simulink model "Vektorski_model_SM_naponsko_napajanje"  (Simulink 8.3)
settings: Solver=ode3  StartTime=0  StopTime=Tfinal  FixedStep=Tsim  RelTol=1e-3
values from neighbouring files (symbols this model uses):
  A1 = [-Rs/Ld 0; 0 -Rs/Lq]    [Vektorski_model_SM_naponsko_napajanje_parametri.m]
  A2 = [0 Lq/Ld; -Ld/Lq 0]    [Vektorski_model_SM_naponsko_napajanje_parametri.m]
  Am = [-Kfv*p/J -Kel*p/J; 1 0]    [Vektorski_model_SM_naponsko_napajanje_parametri.m]
  B = [1/Ld 0; 0 1/Lq]    [Vektorski_model_SM_naponsko_napajanje_parametri.m]
  Bm = [p/J -p/J; 0 0]    [Vektorski_model_SM_naponsko_napajanje_parametri.m]
  Ids_ref = 0    [Vektorski_model_SM_naponsko_napajanje_parametri.m]
  Iqs_ref = 1    [Vektorski_model_SM_naponsko_napajanje_parametri.m]
  Ki = lambda*Rs    [Vektorski_model_SM_naponsko_napajanje_parametri.m]
  Kpd = lambda*Ld    [Vektorski_model_SM_naponsko_napajanje_parametri.m]
  Kpq = lambda*Lq    [Vektorski_model_SM_naponsko_napajanje_parametri.m]
  L = [Ld 0; 0 Lq]    [Vektorski_model_SM_naponsko_napajanje_parametri.m]
  Ld = 0.0370    (= 0.037)    [Vektorski_model_SM_naponsko_napajanje_parametri.m]
  Lq = 0.0485    [Vektorski_model_SM_naponsko_napajanje_parametri.m]
  Mopt = 2    [Vektorski_model_SM_naponsko_napajanje_parametri.m]
  p = 5    [Vektorski_model_SM_naponsko_napajanje_parametri.m]
  PSI = 0.1345    [Vektorski_model_SM_naponsko_napajanje_parametri.m]
  topt = 1    [Vektorski_model_SM_naponsko_napajanje_parametri.m]
  Tsim = Tpwm/16    (= 3.125e-06)    [Vektorski_model_SM_naponsko_napajanje_parametri.m]
libraries: simulink x1

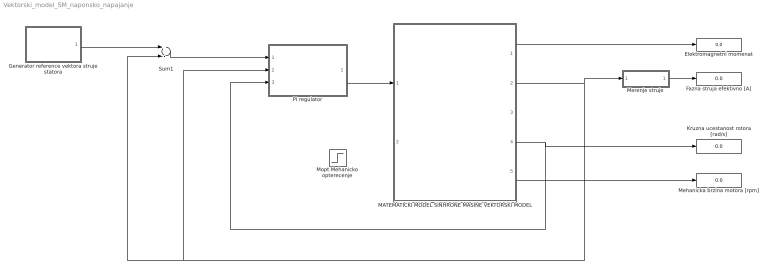
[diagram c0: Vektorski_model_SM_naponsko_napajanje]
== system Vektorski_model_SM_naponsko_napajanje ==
  Elektromagnetni momenat : Display
  Fazna struja efektivno [A] : Display
  Generator reference vektora struje statora : Subsystem
  Kruzna ucestanost rotora [rad/s] : Display
  MATEMATICKI MODEL SINHRONE MASINE VEKTORSKI MODEL : Subsystem
  Mehanicka brzina motora [rpm] : Display
  Merenje struje : Subsystem
  Mopt Mehanicko opterecenje : Step  Time=4*topt  After=Mopt  SampleTime=Tsim
  PI regulator : Subsystem
  Sum1 : Sum  Inputs=+-  SampleTime=Tsim
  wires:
  MATEMATICKI MODEL SINHRONE MASINE VEKTORSKI MODEL/1(M_el) -> Elektromagnetni momenat/1
  MATEMATICKI MODEL SINHRONE MASINE VEKTORSKI MODEL/5(Brzina meh [o/min]) -> Mehanicka brzina motora [rpm]/1
  Merenje struje/1(Is_eff) -> Fazna struja efektivno [A]/1
  MATEMATICKI MODEL SINHRONE MASINE VEKTORSKI MODEL/4(wr_el) -> PI regulator/3(w), Kruzna ucestanost rotora [rad/s]/1
  MATEMATICKI MODEL SINHRONE MASINE VEKTORSKI MODEL/2(Is) -> Merenje struje/1(Is_dq), Sum1/2, PI regulator/2(Is)
  Sum1/1 -> PI regulator/1(e)
  PI regulator/1(Us_ref) -> MATEMATICKI MODEL SINHRONE MASINE VEKTORSKI MODEL/1(Us_dq)
  Generator reference vektora struje statora/1(Is_ref) -> Sum1/1

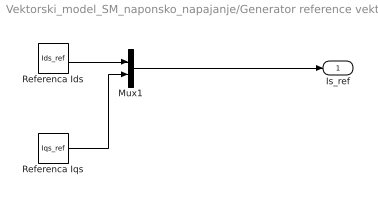
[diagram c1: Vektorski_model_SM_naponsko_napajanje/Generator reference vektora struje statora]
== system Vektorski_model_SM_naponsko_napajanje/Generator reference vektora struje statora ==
  Mux1 : Mux  Inputs=2
  Referenca Ids : Constant  Value=Ids_ref  SampleTime=Tsim
  Referenca Iqs : Constant  Value=Iqs_ref  SampleTime=Tsim
  Is_ref : Outport
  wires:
  Mux1/1 -> Is_ref/1
  Referenca Ids/1 -> Mux1/1
  Referenca Iqs/1 -> Mux1/2

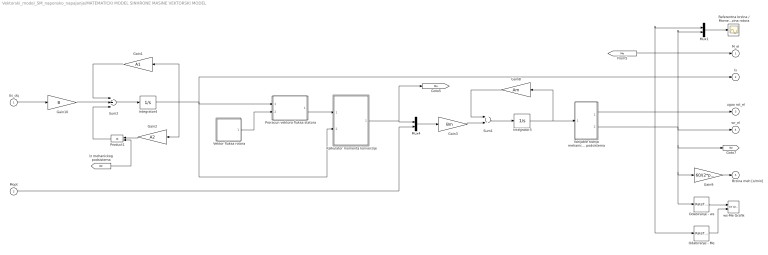
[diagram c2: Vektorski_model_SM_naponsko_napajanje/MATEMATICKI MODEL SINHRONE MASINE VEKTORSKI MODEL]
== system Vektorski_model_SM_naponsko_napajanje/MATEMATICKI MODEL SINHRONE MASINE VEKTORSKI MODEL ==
  Us_dq : Inport
  Mopt : Inport  Port=2
  Gain1 : Gain  Gain=A1  Multiplication=Matrix(K*u) (u vector)  SampleTime=Tsim
  Gain10 : Gain  Gain=B  Multiplication=Matrix(K*u) (u vector)  SampleTime=Tsim
  Gain2 : Gain  Gain=A2  Multiplication=Matrix(K*u) (u vector)  SampleTime=Tsim
  Gain3 : Gain  Gain=Bm  Multiplication=Matrix(K*u) (u vector)  SampleTime=Tsim
  Gain8 : Gain  Gain=Am  Multiplication=Matrix(K*u) (u vector)  SampleTime=Tsim
  Gain9 : Gain  Gain=60/(2*pi()*p)  SampleTime=Tsim
  Integrator3 : Integrator  InitialCondition=[0,0]
  Integrator4 : Integrator  InitialCondition=[0,0]
  Kalkulator momenta konverzije : Subsystem
  Mux1 : Mux  Inputs=2
  Mux4 : Mux  Inputs=2
  Odabiranje - Me : RateTransition  OutPortSampleTime=100*Tsim
  Odabiranje - ws : RateTransition  OutPortSampleTime=100*Tsim
  Product1 : Product  SampleTime=Tsim
  Proracun vektora fluksa statora : Subsystem
  Referentna brzina / Momenat / Brzina rotora : Scope
  Sum1 : Sum  SampleTime=Tsim
  Sum2 : Sum  Inputs=+++  SampleTime=Tsim
  Varijable stanja mehanickog podsistema : Subsystem
  Vektor fluksa rotora : Subsystem
  ws-Me Grafik : simulink/Sinks/XY Graph  xmin=-400  xmax=400  ymin=-20  ymax=20  st=100*Tsim
  M_el : Outport  InitialOutput=0
  Is : Outport  Port=2  InitialOutput=0
  ugao rot_el : Outport  Port=3  InitialOutput=0
  wr_el : Outport  Port=4  InitialOutput=0
  Brzina meh [o/min] : Outport  Port=5  InitialOutput=0
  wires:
  Kalkulator momenta konverzije/1(Me) -> [Me], Mux4/1
  Mopt/1 -> Mux4/2
  [Me] -> Mux1/1, M_el/1, Odabiranje - Me/1
  Varijable stanja mehanickog podsistema/1(theta) -> ugao rot_el/1
  Varijable stanja mehanickog podsistema/2(w) -> Mux1/2, Odabiranje - ws/1, Gain9/1, [Wr], wr_el/1
  Gain9/1 -> Brzina meh [o/min]/1
  Mux4/1 -> Gain3/1
  Gain3/1 -> Sum1/2
  Sum1/1 -> Integrator3/1
  Gain8/1 -> Sum1/1
  Integrator3/1 -> Varijable stanja mehanickog podsistema/1(X2), Gain8/1
  Mux1/1 -> Referentna brzina / Momenat / Brzina rotora/1
  Odabiranje - ws/1 -> ws-Me Grafik/1
  Odabiranje - Me/1 -> ws-Me Grafik/2
  Sum2/1 -> Integrator4/1
  Gain2/1 -> Product1/1
  Integrator4/1 -> Kalkulator momenta konverzije/2(Is), Is/1, Proracun vektora fluksa statora/1(Is), Gain2/1, Gain1/1
  [Wr] -> Product1/2
  Gain1/1 -> Sum2/1
  Product1/1 -> Sum2/3
  Gain10/1 -> Sum2/2
  Us_dq/1 -> Gain10/1
  Proracun vektora fluksa statora/1(PSIs) -> Kalkulator momenta konverzije/1(PSIs)
  Vektor fluksa rotora/1("[PSIpm 0]") -> Proracun vektora fluksa statora/2(PSIr)

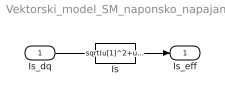
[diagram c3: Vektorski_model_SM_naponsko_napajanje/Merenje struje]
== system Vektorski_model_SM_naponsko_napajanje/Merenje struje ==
  Is_dq : Inport
  Is : Fcn  Expr=sqrt(u[1]^2+u[2]^2)  SampleTime=Tsim
  Is_eff : Outport
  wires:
  Is_dq/1 -> Is/1
  Is/1 -> Is_eff/1

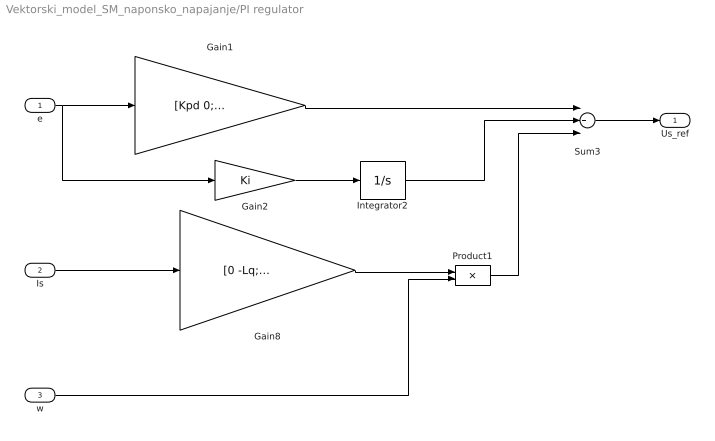
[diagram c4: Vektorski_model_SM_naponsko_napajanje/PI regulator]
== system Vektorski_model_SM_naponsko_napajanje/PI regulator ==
  e : Inport
  Is : Inport  Port=2
  w : Inport  Port=3
  Gain1 : Gain  Gain=[Kpd 0; 0 Kpq]  Multiplication=Matrix(K*u) (u vector)  SampleTime=Tsim
  Gain2 : Gain  Gain=Ki  SampleTime=Tsim
  Gain8 : Gain  Gain=[0 -Lq; Ld 0]  Multiplication=Matrix(K*u) (u vector)  SampleTime=Tsim
  Integrator2 : Integrator  InitialCondition=[0,0]
  Product1 : Product  SampleTime=Tsim
  Sum3 : Sum  Inputs=+++  SampleTime=Tsim
  Us_ref : Outport
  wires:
  Sum3/1 -> Us_ref/1
  Gain2/1 -> Integrator2/1
  Integrator2/1 -> Sum3/2
  e/1 -> Gain2/1, Gain1/1
  Gain1/1 -> Sum3/1
  Is/1 -> Gain8/1
  Gain8/1 -> Product1/1
  w/1 -> Product1/2
  Product1/1 -> Sum3/3

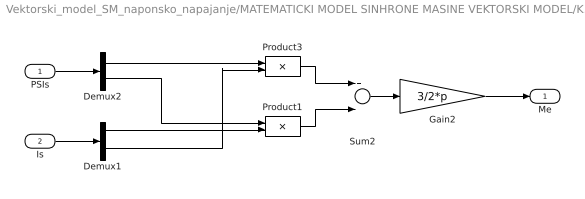
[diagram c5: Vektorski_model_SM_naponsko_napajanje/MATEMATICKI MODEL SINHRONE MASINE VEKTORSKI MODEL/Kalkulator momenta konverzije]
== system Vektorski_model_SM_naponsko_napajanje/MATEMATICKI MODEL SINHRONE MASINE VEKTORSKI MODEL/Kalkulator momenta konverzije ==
  PSIs : Inport
  Is : Inport  Port=2
  Demux1 : Demux  Outputs=2
  Demux2 : Demux  Outputs=2
  Gain2 : Gain  Gain=3/2*p  SampleTime=Tsim
  Product1 : Product  SampleTime=Tsim
  Product3 : Product  SampleTime=Tsim
  Sum2 : Sum  Inputs=+-  SampleTime=Tsim
  Me : Outport
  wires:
  Sum2/1 -> Gain2/1
  Gain2/1 -> Me/1
  Product1/1 -> Sum2/2
  Product3/1 -> Sum2/1
  Demux2/1 -> Product3/1
  Demux2/2 -> Product1/1
  Is/1 -> Demux1/1
  Demux1/2 -> Product3/2
  Demux1/1 -> Product1/2
  PSIs/1 -> Demux2/1

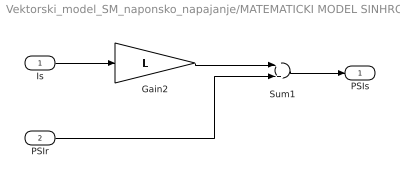
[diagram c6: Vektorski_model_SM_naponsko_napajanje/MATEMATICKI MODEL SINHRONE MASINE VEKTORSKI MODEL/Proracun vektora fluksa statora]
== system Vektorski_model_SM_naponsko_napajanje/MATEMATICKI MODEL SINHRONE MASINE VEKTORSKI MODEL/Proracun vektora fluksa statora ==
  Is : Inport
  PSIr : Inport  Port=2
  Gain2 : Gain  Gain=L  Multiplication=Matrix(K*u) (u vector)  SampleTime=Tsim
  Sum1 : Sum  SampleTime=Tsim
  PSIs : Outport
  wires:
  Sum1/1 -> PSIs/1
  Gain2/1 -> Sum1/1
  PSIr/1 -> Sum1/2
  Is/1 -> Gain2/1

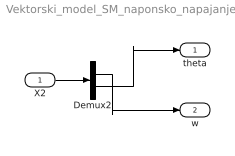
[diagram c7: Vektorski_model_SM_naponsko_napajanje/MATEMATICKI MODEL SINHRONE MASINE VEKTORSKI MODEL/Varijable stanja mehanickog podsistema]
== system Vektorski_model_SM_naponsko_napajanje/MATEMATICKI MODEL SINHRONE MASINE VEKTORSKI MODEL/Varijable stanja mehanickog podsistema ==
  X2 : Inport
  Demux2 : Demux  Outputs=2
  theta : Outport
  w : Outport  Port=2
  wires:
  X2/1 -> Demux2/1
  Demux2/2 -> theta/1
  Demux2/1 -> w/1

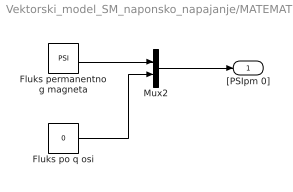
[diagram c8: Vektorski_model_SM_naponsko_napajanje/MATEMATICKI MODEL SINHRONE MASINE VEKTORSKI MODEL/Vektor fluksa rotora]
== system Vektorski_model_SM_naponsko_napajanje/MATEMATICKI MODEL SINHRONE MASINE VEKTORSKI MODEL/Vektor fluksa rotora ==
  Fluks permanentnog magneta : Constant  Value=PSI  SampleTime=Tsim
  Fluks po q osi : Constant  Value=0  SampleTime=Tsim
  Mux2 : Mux  Inputs=2
  "[PSIpm 0]" : Outport
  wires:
  Fluks permanentnog magneta/1 -> Mux2/1
  Fluks po q osi/1 -> Mux2/2
  Mux2/1 -> "[PSIpm 0]"/1
